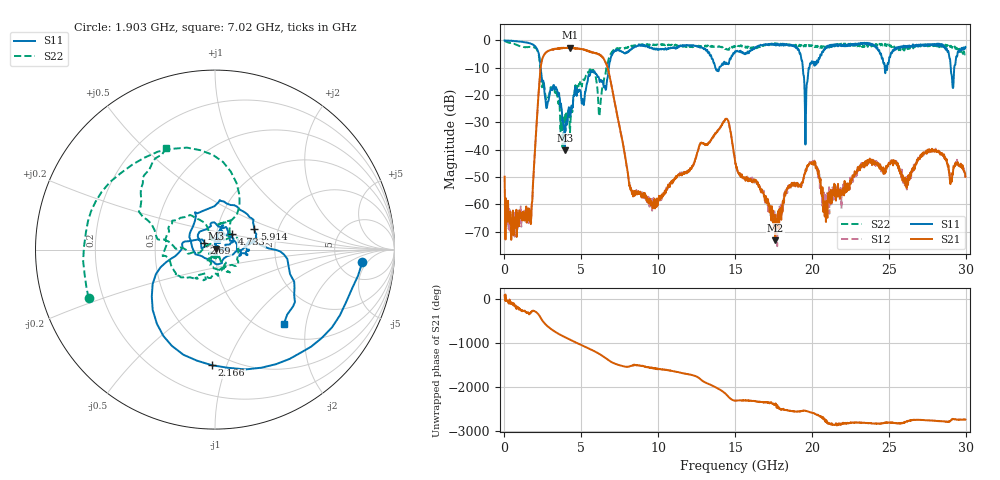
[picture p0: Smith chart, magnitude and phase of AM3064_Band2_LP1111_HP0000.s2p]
# Hz S DB R 50.0
!freq dBS11 angS11 dBS21 angS21 dBS12 angS12 dBS22 angS22
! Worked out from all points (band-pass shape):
!   1600 points, 10 MHz to 29.98 GHz, reference 50 ohm
!   highest |S21| = -2.68 dB at 4.246 GHz (marker M1); lowest = -73.1 dB at 17.61 GHz (marker M2)
!   |S21| within 3 dB of the highest: 2.544 GHz to 6.298 GHz (3.754 GHz wide, 84.9 % of centre)
!   lowest |S11| = -40.2 dB at 3.927 GHz (marker M3), VSWR 1.02, Z = 50.8 + j0.595 ohm
!   |S11| at or under -10 dB: 2.354 GHz to 6.784 GHz (4.43 GHz wide, 97 % of centre); 13.72 GHz to 13.97 GHz (258.1 MHz wide, 1.86 % of centre); 19.41 GHz to 19.83 GHz (426.6 MHz wide, 2.17 % of centre)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
!   |S22| runs from -39.1 to -0.1 dB; largest |S21 - S12| = 0.016
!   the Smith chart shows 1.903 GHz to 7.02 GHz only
!   S11 on the Smith chart (normalised r, x): 1.903 GHz: 8.74, -3.77; 2.166 GHz: 0.40, -0.89; 2.69 GHz: 0.89, +0.07; 4.733 GHz: 1.19, +0.21; 5.914 GHz: 1.50, +0.37; 7.02 GHz: 1.24, -1.50
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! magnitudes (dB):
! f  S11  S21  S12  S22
! 10 MHz  0.0  -49.9  -60.4  -0.1
! 1.603 GHz  -1.0  -62.0  -62.9  -2.4
! 1.903 GHz  -1.7  -48.2  -48.0  -2.5
! 2.166 GHz  -3.8  -23.7  -23.7  -4.0
! 2.69 GHz  -23.0  -4.5  -4.5  -21.5
! 3.927 GHz  -40.2  -2.7  -2.7  -29.7
! 4.246 GHz  -25.2  -2.7  -2.7  -33.1
! 4.733 GHz  -17.9  -2.9  -2.9  -17.0
! 5.015 GHz  -22.2  -3.1  -3.1  -16.2
! 5.914 GHz  -12.1  -4.6  -4.7  -12.7
! 7.02 GHz  -5.0  -18.2  -18.1  -4.0
! 8.257 GHz  -3.1  -55.1  -54.2  -1.9
! 10 GHz  -3.3  -58.0  -58.1  -1.7
! 14.37 GHz  -8.6  -28.8  -28.8  -3.2
! 15 GHz  -4.1  -44.1  -44.0  -2.2
! 17.61 GHz  -1.6  -73.1  -65.9  -1.1
! 19.11 GHz  -3.3  -53.5  -53.3  -2.2
! 19.58 GHz  -38.1  -48.1  -47.3  -2.1
! 19.99 GHz  -7.6  -44.6  -44.7  -1.8
! 20.87 GHz  -2.8  -62.0  -56.5  -2.8
! 25 GHz  -8.0  -44.8  -45.1  -1.5
! 29.98 GHz  -2.4  -49.9  -50.2  -4.4
